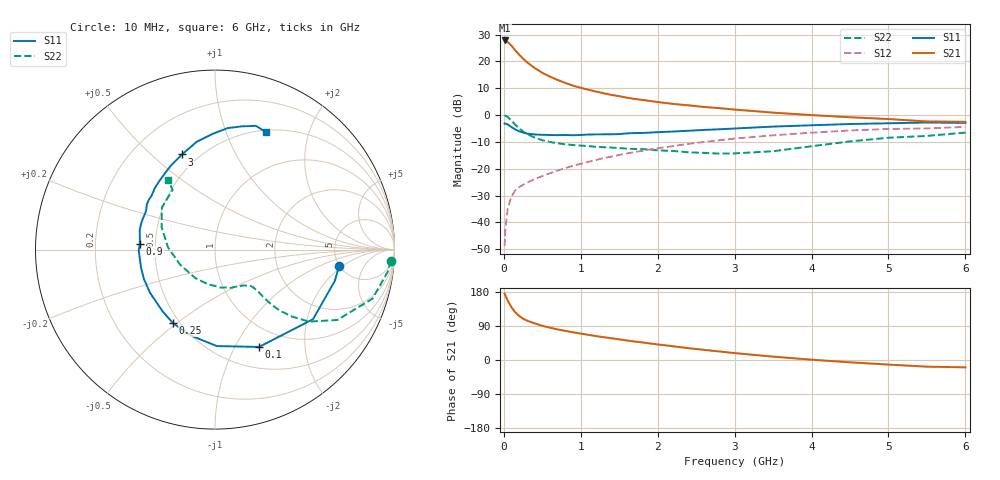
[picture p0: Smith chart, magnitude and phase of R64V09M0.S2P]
! SIEMENS Small Signal Semiconductors
! BFR193
! Si NPN RF Bipolar Junction Transistor in SOT23
! VCE = 4 V  IC = 9 mA
! Common Emitter S-Parameters:  May  1996
# GHz  S  MA  R  50
!  f  S11  S21  S12  S22
! GHz  MAG  ANG  MAG  ANG  MAG  ANG  MAG  ANG
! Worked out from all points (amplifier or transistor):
!   36 points, 10 MHz to 6 GHz, reference 50 ohm
!   highest |S21| = 27.8 dB at 10 MHz (marker M1)
!   |S21| within 3 dB of that: start of sweep to 129 MHz
!   unconditionally stable (mu >= 1): 760.9 MHz to 1.982 GHz
!   at 250 MHz: K = 0.61, MSG = 23.5 dB, |S12| = -26.0 dB
!   at 1.4 GHz: K = 1.05, MAG = 10.1 dB, |S12| = -15.5 dB
!   at 6 GHz: K = 0.95, MSG = 0.9 dB, |S12| = -4.4 dB
!   S11 on the Smith chart (normalised r, x): 10 MHz: 4.97, -1.76; 100 MHz: 0.75, -1.26; 250 MHz: 0.46, -0.48; 900 MHz: 0.41, +0.03; 3 GHz: 0.41, +0.63; 6 GHz: 0.53, +1.40
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0.01  0.6977 -7.5  24.55 175.3  0.0036 83.6  0.9821 -3.6
0.02  0.6899 -14.7  24.29 170.2  0.0076 79.5  0.9705 -7.3
0.05  0.6696 -35.4  22.96 157.0  0.0179 74.1  0.919 -17.3
0.1  0.5953 -65.6  19.55 138.8  0.0308 63.9  0.7864 -29.9
0.15  0.5377 -88.9  15.97 125.3  0.0396 57.3  0.6589 -37.5
0.2  0.497 -106.2  13.32 116.2  0.0455 55.0  0.5661 -41.1
0.25  0.4716 -119.8  11.25 109.1  0.0501 54.2  0.4939 -43.3
0.3  0.4512 -130.3  9.67 104.0  0.0547 55.0  0.4429 -44.2
0.4  0.4347 -146.1  7.533 96.6  0.0641 55.9  0.3804 -44.5
0.5  0.4287 -157.2  6.122 90.2  0.0729 57.7  0.3397 -44.2
0.6  0.4243 -165.9  5.185 85.2  0.0823 59.4  0.3136 -44.4
0.7  0.422 -173.5  4.499 80.6  0.0922 60.9  0.2974 -44.7
0.9  0.4201 175.4  3.535 73.1  0.1135 61.6  0.276 -46.0
1.1  0.4331 165.7  2.96 66.3  0.1347 62.2  0.2632 -49.5
1.3  0.4372 157.3  2.537 60.1  0.1574 61.7  0.2509 -53.1
1.6  0.4554 146.6  2.105 51.5  0.1924 60.1  0.2365 -61.0
2.2  0.4927 128.8  1.611 36.2  0.2647 54.9  0.2141 -81.3
3  0.561 109.1  1.265 18.2  0.3641 44.5  0.193 -124.4
3.5  0.6095 99.6  1.11 8.9  0.4189 37.0  0.2116 -156.3
4.5  0.6808 84.0  0.91 -6.1  0.5159 21.8  0.3225 157.3
5.5  0.7261 71.7  0.76 -17.6  0.5628 6.1  0.4084 125.3
6  0.7133 66.3  0.748 -19.4  0.6015 1.5  0.4703 124.1
